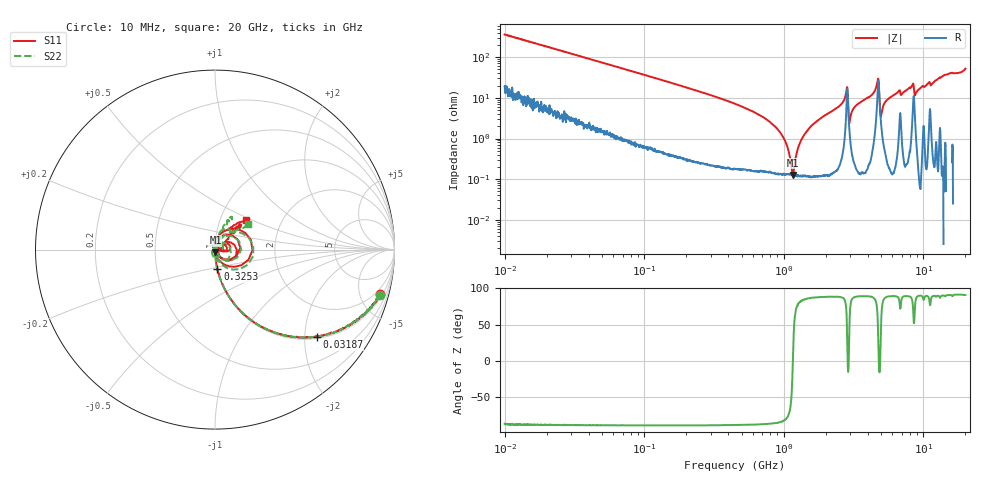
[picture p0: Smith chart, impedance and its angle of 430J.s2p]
!Keysight Technologies,P5008B,MY61100088,A.16.20.02
!Date: Tuesday, November 07, 2023 16:23:38
!Correction: S11(C  2-Port  )
!S21(C  2-Port  )
!S12(C  2-Port  )
!S22(C  2-Port  )
!S2P File: Measurements: S11, S21, S12, S22:Log Frequency Sweep
# Hz S  dB  R 50
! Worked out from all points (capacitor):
!   1601 points, 10 MHz to 20 GHz, reference 50 ohm
!   read as one part in series: C = 44 pF near 10.39 MHz
!   lowest |Z| = 126 mohm at 1.162 GHz (marker M1)
!   series resonance near 1.161 GHz, so ESL is about 430 pH
!   S11 on the Smith chart (normalised r, x): 10 MHz: 1.37, -7.21; 31.87 MHz: 1.05, -2.29; 325.3 MHz: 1.00, -0.22; 20 GHz: 1.33, +0.46
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1e7  -0.44 -15.2  -11.59 71.7  -11.59 71.8  -0.43 -15.3
3.187184e7  -2.55 -40.6  -3.73 48.2  -3.74 48.2  -2.55 -40.7
3.555162e7  -2.99 -43.6  -3.23 45.1  -3.23 45.1  -2.99 -43.6
1.263918e8  -11.09 -73.0  -0.39 16.0  -0.39 16.0  -11.09 -73.2
3.253002e8  -19.22 -82.9  -0.07 5.8  -0.07 5.8  -19.21 -83.4
4.472136e8  -22.24 -84.6  -0.04 3.7  -0.04 3.7  -22.24 -85.2
1.162002e9  -36.45 -81.0  -0.01 -0.9  -0.01 -0.9  -36.44 -90.5
1.411873e9  -43.80 -61.6  -0.01 -1.8  -0.01 -1.8  -44.59 -98.1
1.589917e9  -49.86 0.4  -0.01 -2.4  -0.01 -2.4  -62.83 -170.5
2.811588e9  -19.43 51.5  -0.54 -9.9  -0.54 -9.9  -19.26 45.3
3.106545e9  -45.81 98.8  -0.03 -5.4  -0.03 -5.4  -40.21 16.4
3.367837e9  -33.15 94.5  -0.01 -6.7  -0.01 -6.7  -33.18 61.1
4.7413e9  -13.67 15.1  -1.87 -13.5  -1.88 -13.5  -13.38 6.0
5.390168e9  -42.42 -71.1  -0.02 -9.9  -0.02 -9.8  -41.67 -47.0
5.652411e9  -45.39 -0.0  0.00 -11.0  -0.00 -11.0  -48.29 45.6
6.70667e9  -25.78 32.3  -0.12 -15.2  -0.13 -15.1  -28.45 68.7
7.133913e9  -29.76 6.7  -0.01 -14.6  -0.01 -14.6  -34.14 126.0
8.5048e9  -18.29 -0.5  -0.89 -19.2  -0.90 -19.2  -20.79 -13.1
9.30816e9  -32.73 -32.9  0.02 -19.4  0.02 -19.4  -36.47 -170.9
9.948277e9  -28.59 13.4  -0.09 -22.0  -0.09 -21.9  -35.61 58.0
1.354728e10  -16.36 47.1  -0.07 -30.3  -0.07 -30.2  -16.51 68.5
2e10  -12.48 43.4  -0.24 -51.4  -0.25 -51.3  -12.60 37.9
